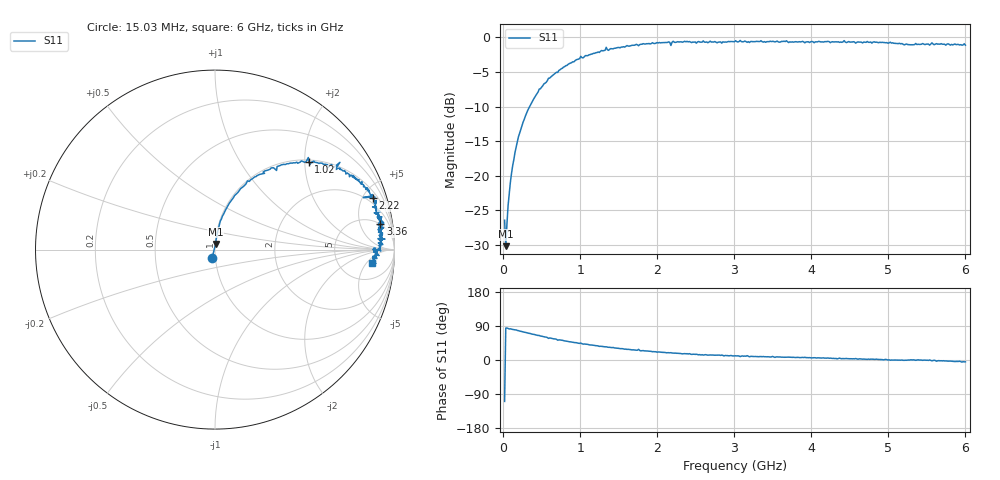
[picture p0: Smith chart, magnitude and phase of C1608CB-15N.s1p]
!	Network	Analyzer	HP8753E.07.74:	Oct	30	2002	Serial	No.	JP38451487
!	Hewlett-Packard
!	7	Sep	2009	9:36:41
!	Frequency	S11
#	HZ	S	RI	R	50
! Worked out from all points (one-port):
!   400 points, 15.03 MHz to 6 GHz, reference 50 ohm
!   lowest |S11| = -30.2 dB at 30.03 MHz (marker M1), VSWR 1.06, Z = 50.2 + j3.1 ohm
!   |S11| at or under -10 dB: start of sweep to 340.4 MHz
!   S11 on the Smith chart (normalised r, x): 15.03 MHz: 0.97, -0.09; 1.02 GHz: 1.05, +2.10; 2.22 GHz: 1.52, +5.92; 3.36 GHz: 5, +11; 6 GHz: 11, -7
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1.502992e7  -0.0157 -0.045
3.002985e7  0.00309 0.0308
6.00297e7  0.00706 0.0603
1.050295e8  0.0157 0.103
1.650292e8  0.0297 0.159
2.550287e8  0.0667 0.235
4.650277e8  0.181 0.383
7.650262e8  0.369 0.472
1.020025e9  0.523 0.487
1.335023e9  0.696 0.486
1.515022e9  0.729 0.421
1.725021e9  0.803 0.389
1.755021e9  0.768 0.412
1.785021e9  0.815 0.365
1.99502e9  0.86 0.324
2.145019e9  0.877 0.307
2.175019e9  0.826 0.29
2.220019e9  0.878 0.286
2.265019e9  0.888 0.284
2.505017e9  0.878 0.238
2.595017e9  0.921 0.211
2.835016e9  0.887 0.205
3.015015e9  0.93 0.182
3.360013e9  0.922 0.142
3.765011e9  0.918 0.116
4.515007e9  0.925 0.0545
5.265004e9  0.887 -0.00388
6e9  0.877 -0.0733
